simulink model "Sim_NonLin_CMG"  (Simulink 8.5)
settings: Solver=ode4  StartTime=0.0  StopTime=1800  FixedStep=Ts*1  RelTol=1e-3
InitFcn:
  | start
StopFcn:
  | Pl2
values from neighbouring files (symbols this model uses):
  Ave = [    [vehicle_flex34.m]    (also in vehicle_rigid.m)
  Bve = [    [vehicle_flex34.m]    (also in vehicle_rigid.m)
  CB2L = [cpsi, -cphi*spsi,  sphi*spsi;          0,    cphi,      -sphi;          0,    sphi*cpsi,  cphi*cpsi]/cpsi    [Rigbod_Dynam_LVLH.m]    (also in start.m = eye(3); start2.m = eye(3); start3.m = eye(3); start1.m = eye(3))
  com_dir = com_dir/sqrt(com_dir'*com_dir)    [start.m]    (also in start2.m; start3.m; start1.m)
  Cve = [    [vehicle_flex34.m]    (also in vehicle_rigid.m)
  d2r = pi/180    (= 0.0174532925199)    [start.m]    (also in start2.m; start3.m; Dead_Band_DF.m; start1.m)
  Dve = [    [vehicle_flex34.m]    (also in vehicle_rigid.m)
  ini = [wbo; atto; Hco]    [start.m]    (also in start2.m; start3.m; start1.m)
  J = [0.119416e9, -0.476e7,   -0.1216e7;     -0.476e7,     0.40408e8, -0.30121e6;     -0.1216e7,   -0.30121e6,  0.110166e9]    [start.m]    (also in start2.m; start3.m; start1.m)
  KshC = 2*Wdot_Lim_CMG/WlimC    [start.m]    (also in start2.m; start3.m; start1.m)
  nt = 12    [start.m]    (also in start2.m; start3.m; start1.m)
  omg = 20*wo    (= 0.022)    [start.m]    (also in start2.m; start3.m; start1.m)
  r2d = 180/pi    (= 57.2957795131)    [start.m]    (also in start2.m; start3.m; start1.m)
  thecmd = 20    [start.m]    (also in start2.m; start3.m; start1.m = 0.1)
  Wdot_Lim_CMG = 0.0001*d2r    (= 1.74532925199e-06)    [start.m]    (also in start2.m; start3.m; start1.m)
  Wlim_CMG = 0.01*d2r    (= 0.000174532925199)    [start.m]    (also in start2.m; start3.m; start1.m)
  wo = 0.0011    [start.m]    (also in start2.m; start3.m; start1.m)
  zeb = 0.95    [start.m]    (also in start2.m; start3.m; start1.m)
undefined symbols (not defined in the file or in its folder): Rigbod_Dynam_LVLH, Torq_Lim, Wlim

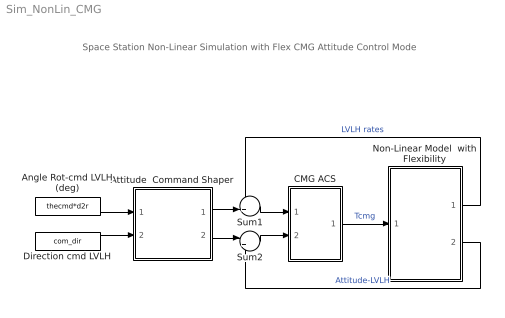
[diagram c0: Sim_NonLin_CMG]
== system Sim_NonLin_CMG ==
  note: Space Station Non-Linear Simulation with Flex CMG Attitude Control Mode
  Angle Rot-cmd LVLH (deg) : Constant  Value=thecmd*d2r
  Attitude  Command Shaper : Subsystem
  CMG ACS : Subsystem
  Direction cmd LVLH : Constant  Value=com_dir
  Non-Linear Model  with Flexibility : Subsystem
  Sum1 : Sum  Inputs=-+|
  Sum2 : Sum  Inputs=|+-
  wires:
  Non-Linear Model  with Flexibility/2(atti) -> Sum2/2  "Attitude-LVLH"
  Sum2/1 -> CMG ACS/2(ater)
  Non-Linear Model  with Flexibility/1(wlv) -> Sum1/1  "LVLH rates"
  Direction cmd LVLH/1 -> Attitude  Command Shaper/2(dir)
  Angle Rot-cmd LVLH (deg)/1 -> Attitude  Command Shaper/1(cmd)
  Sum1/1 -> CMG ACS/1(wl)
  CMG ACS/1(Tq) -> Non-Linear Model  with Flexibility/1(Tcmg)  "Tcmg"
  Attitude  Command Shaper/2(att-cmd) -> Sum2/1
  Attitude  Command Shaper/1(w-cmd) -> Sum1/2

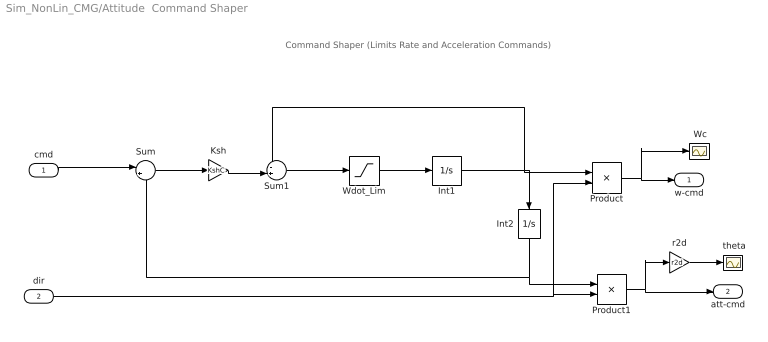
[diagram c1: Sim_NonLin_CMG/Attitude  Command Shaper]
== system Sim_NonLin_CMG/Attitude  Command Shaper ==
  note: Command Shaper (Limits Rate and Acceleration Commands)
  cmd : Inport  PortDimensions=1
  dir : Inport  Port=2  PortDimensions=3
  " Wc" : Scope
  " theta" : Scope
  Int1 : Integrator  LimitOutput=on  UpperSaturationLimit=Wlim_CMG  LowerSaturationLimit=-Wlim_CMG
  Int2 : Integrator  UpperSaturationLimit=Wlim  LowerSaturationLimit=-Wlim
  Ksh : Gain  Gain=KshC
  Product : Product
  Product1 : Product
  Sum : Sum  Inputs=|+-
  Sum1 : Sum  Inputs=-+|
  Wdot_Lim : Saturate  UpperLimit=Wdot_Lim_CMG  LowerLimit=-Wdot_Lim_CMG
  r2d : Gain  Gain=r2d
  w-cmd : Outport  PortDimensions=3
  att-cmd : Outport  Port=2  PortDimensions=3
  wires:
  Wdot_Lim/1 -> Int1/1
  Sum1/1 -> Wdot_Lim/1
  Int1/1 -> Product/1, Sum1/1, Int2/1
  Sum/1 -> Ksh/1
  Ksh/1 -> Sum1/2
  Int2/1 -> Sum/2, Product1/1
  cmd/1 -> Sum/1
  dir/1 -> Product/2, Product1/2
  r2d/1 -> " theta"/1
  Product/1 -> w-cmd/1, " Wc"/1
  Product1/1 -> att-cmd/1, r2d/1

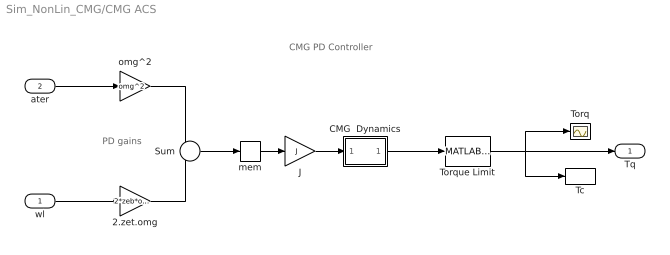
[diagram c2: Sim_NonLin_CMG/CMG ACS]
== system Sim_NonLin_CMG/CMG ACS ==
  note: CMG PD Controller
  note: PD gains
  wl : Inport
  ater : Inport  Port=2  PortDimensions=3
  2.zet.omg : Gain  Gain=2*zeb*omg
  CMG  Dynamics : Subsystem
  J : Gain  Gain=J  Multiplication=Matrix(K*u)
  Sum : Sum  Inputs=--
  Tc : ToWorkspace  VariableName=Tcmg  SampleTime=-1
  Torq : Scope
  Torque Limit : MATLABFcn  MATLABFcn=Torq_Lim( u(1:3) )  OutputDimensions=3
  mem : Memory
  omg^2 : Gain  Gain=omg^2
  Tq : Outport
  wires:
  wl/1 -> 2.zet.omg/1
  Sum/1 -> mem/1
  2.zet.omg/1 -> Sum/2
  ater/1 -> omg^2/1
  omg^2/1 -> Sum/1
  J/1 -> CMG  Dynamics/1(I)
  mem/1 -> J/1
  Torque Limit/1 -> Tq/1, Torq/1, Tc/1
  CMG  Dynamics/1(O) -> Torque Limit/1

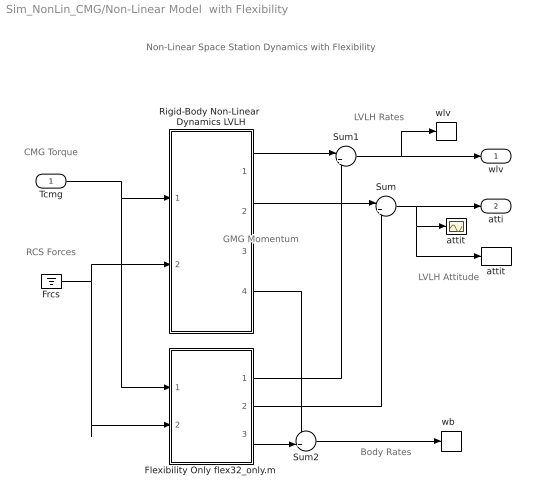
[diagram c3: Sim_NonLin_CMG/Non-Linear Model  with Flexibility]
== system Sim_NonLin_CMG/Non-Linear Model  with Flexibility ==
  note: Non-Linear Space Station Dynamics with Flexibility
  note: LVLH Attitude
  note: Body Rates
  note: RCS Forces
  note: CMG Torque
  note: LVLH Rates
  note: GMG Momentum
  Tcmg : Inport
  " attit " : Scope
  Flexibility Only flex32_only.m : Subsystem
  Frcs : Ground
  Rigid-Body Non-Linear  Dynamics LVLH : Subsystem
  Sum : Sum  Inputs=|++
  Sum1 : Sum  Inputs=|++
  Sum2 : Sum  Inputs=++|
  attit : ToWorkspace  VariableName=theta  SampleTime=-1
  "wb  " : ToWorkspace  VariableName=wb  SampleTime=-1
  "wlv  " : ToWorkspace  VariableName=wl  SampleTime=-1
  wlv : Outport
  atti : Outport  Port=2
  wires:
  Frcs/1 -> Rigid-Body Non-Linear  Dynamics LVLH/2(Frcs), Flexibility Only flex32_only.m/2(Frcs)
  Rigid-Body Non-Linear  Dynamics LVLH/2(atti-lv) -> Sum/1
  Flexibility Only flex32_only.m/2(att) -> Sum/2
  Sum/1 -> atti/1, " attit "/1, attit/1
  Sum1/1 -> wlv/1, "wlv  "/1
  Tcmg/1 -> Rigid-Body Non-Linear  Dynamics LVLH/1(Tcmg), Flexibility Only flex32_only.m/1(Tcmg)
  Rigid-Body Non-Linear  Dynamics LVLH/1(w-lv) -> Sum1/1
  Flexibility Only flex32_only.m/1(wbf) -> Sum1/2
  Flexibility Only flex32_only.m/3(wb) -> Sum2/2
  Rigid-Body Non-Linear  Dynamics LVLH/4(wb) -> Sum2/1
  Sum2/1 -> "wb  "/1

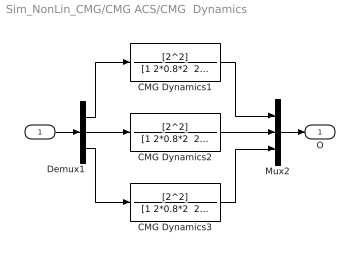
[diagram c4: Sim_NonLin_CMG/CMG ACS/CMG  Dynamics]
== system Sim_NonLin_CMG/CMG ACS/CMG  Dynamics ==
  I : Inport
  CMG Dynamics1 : TransferFcn  Numerator=[2^2]  Denominator="[1 2*0.8*2  2^2]"
  CMG Dynamics2 : TransferFcn  Numerator=[2^2]  Denominator="[1 2*0.8*2  2^2]"
  CMG Dynamics3 : TransferFcn  Numerator=[2^2]  Denominator="[1 2*0.8*2  2^2]"
  Demux1 : Demux  Outputs=3
  Mux2 : Mux  Inputs=3
  O : Outport
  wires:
  Mux2/1 -> O/1
  I/1 -> Demux1/1
  Demux1/3 -> CMG Dynamics3/1
  Demux1/1 -> CMG Dynamics1/1
  Demux1/2 -> CMG Dynamics2/1
  CMG Dynamics1/1 -> Mux2/1
  CMG Dynamics3/1 -> Mux2/3
  CMG Dynamics2/1 -> Mux2/2

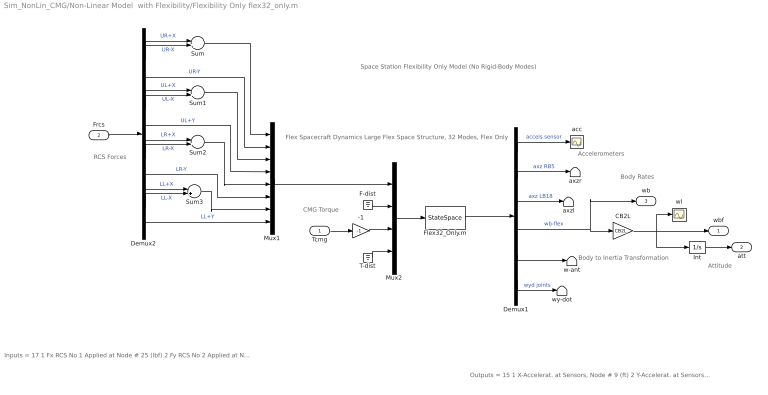
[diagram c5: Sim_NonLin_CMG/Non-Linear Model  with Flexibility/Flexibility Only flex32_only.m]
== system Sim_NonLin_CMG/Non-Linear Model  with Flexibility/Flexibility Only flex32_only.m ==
  note: Space Station Flexibility Only Model (No Rigid-Body Modes)
  note: Body to Inertia Transformation
  note: Attitude
  note: Body Rates
  note: Accelerometers
  note: Flex Spacecraft Dynamics Large Flex Space Structure, 32 Modes, Flex Only
  note: CMG Torque
  note: RCS Forces
  note: Inputs = 17 1 Fx RCS No 1 Applied at Node # 25 (lbf) 2 Fy RCS No 2 Applied at Node # 25 (lbf) 3 Fx RCS No 3 Applied at Node # 26 (lbf) 4 Fy RCS No 4 Applied at Node # 26 (lbf) 5 Fx RCS No 5 Applied at Node # 27 (lbf) 6 Fy RCS No 6 Applied at Node # 27 (lbf) 7 Fx RCS No 7 Applied at Node # 28 (lbf) 8 Fy RCS No 8 Applied at Node # 28 (lbf) 9 Fx Disturb. No 9 at Node # 21 (lbf) 10 Fy Disturb. No 10 at Node # 21 (lbf) 11 Fz Disturb. No 11 at Node # 21 (lbf) 12 Torq-x No 1 CMG Applied at Node # 10 (ft-lb) 13 Torq-y No 2 CMG Applied at Node # 10 (ft-lb) 14 Torq-z No 3 CMG Applied at Node # 10 (ft-lb) 15 Torq-x No 4 Gimbal Dist. at Node # 1 (ft-lb) 16 Torq-y No 5 Gimbal Dist. at Node # 1 (ft-lb) 17 Torq-z No 6 Gimbal Dist. at Node # 1 (ft-lb)
  note: Outputs = 15 1 X-Accelerat. at Sensors, Node # 9 (ft) 2 Y-Accelerat. at Sensors, Node # 9 (ft) 3 Z-Accelerat. at Sensors, Node # 9 (ft) 4 X-Accelerat. at Right Boom End, Node # 5 (ft) 5 Z-Accelerat. at Right Boom End, Node # 5 (ft) 6 X-Accelerat. at Left Boom End, Node # 18 (ft) 7 Z-Accelerat. at Left Boom End, Node # 18 (ft) 8 X-Rot. Rate at Sensors, Node # 9 (radian) 9 Y-Rot. Rate at Sensors, Node # 9 (radian) 10 Z-Rot. Rate at Sensors, Node # 9 (radian) 11 X-Rot. Rate at Antena Bot-Left, Node # 24 (radian) 12 Y-Rot. Rate at Antena Bot-Left, Node # 24 (radian) 13 Z-Rot. Rate at Antena Bot-Left, Node # 24 (radian) 14 Y-Rot.Accel. at Right Joint, Node # 7 (radian) 15 Y-Rot.Accel. at Left Joint, Node # 16 (radian)
  Tcmg : Inport
  Frcs : Inport  Port=2
  -1 : Gain  Gain=-1
  CB2L : Gain  Gain=CB2L  Multiplication=Matrix(K*u)
  Demux1 : Demux  Outputs=[3, 2, 2, 3, 3, 2]
  Demux2 : Demux  Outputs=12
  F-dist : Ground
  Flex32_Only.m : StateSpace  A=Ave  B=Bve  C=Cve  D=Dve  X0=0
  Int : Integrator
  Mux1 : Mux  Inputs=8
  Mux2 : Mux  Inputs=[8, 3, 3, 3]
  Sum{,1..3} (4 alike) : Sum  Inputs=|+-
  T-dist : Ground
  acc : Scope
  axzl : Terminator
  axzr : Terminator
  w-ant : Terminator
  wl : Scope
  wy-dot : Terminator
  wbf : Outport
  att : Outport  Port=2
  wb : Outport  Port=3
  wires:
  Demux1/6 -> wy-dot/1  "wyd joints"
  Demux1/5 -> w-ant/1
  T-dist/1 -> Mux2/4
  F-dist/1 -> Mux2/2
  Demux1/3 -> axzl/1  "axz LB18"
  Demux1/2 -> axzr/1  "axz RB5"
  Tcmg/1 -> -1/1
  Demux1/4 -> CB2L/1, wb/1  "wb-flex"
  Demux1/1 -> acc/1  "accels sensor"
  Flex32_Only.m/1 -> Demux1/1
  Mux2/1 -> Flex32_Only.m/1
  Mux1/1 -> Mux2/1
  Frcs/1 -> Demux2/1
  Demux2/6 -> Mux1/4  "UL+Y"
  Demux2/9 -> Mux1/6  "LR-Y"
  Demux2/12 -> Mux1/8  "LL+Y"
  Demux2/3 -> Mux1/2  "UR-Y"
  Demux2/1 -> Sum/1  "UR+X"
  Demux2/2 -> Sum/2  "UR-X"
  Sum/1 -> Mux1/1
  Demux2/4 -> Sum1/1  "UL+X"
  Demux2/5 -> Sum1/2  "UL-X"
  Sum1/1 -> Mux1/3
  Demux2/7 -> Sum2/1  "LR+X"
  Demux2/8 -> Sum2/2  "LR-X"
  Demux2/10 -> Sum3/1  "LL+X"
  Demux2/11 -> Sum3/2  "LL-X"
  Sum3/1 -> Mux1/7
  Sum2/1 -> Mux1/5
  Int/1 -> att/1
  -1/1 -> Mux2/3
  CB2L/1 -> wl/1, wbf/1, Int/1

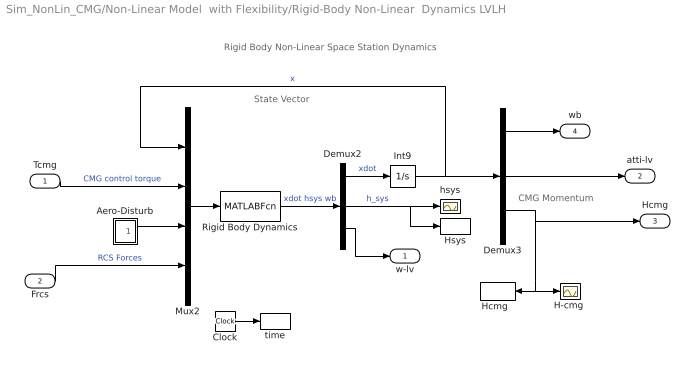
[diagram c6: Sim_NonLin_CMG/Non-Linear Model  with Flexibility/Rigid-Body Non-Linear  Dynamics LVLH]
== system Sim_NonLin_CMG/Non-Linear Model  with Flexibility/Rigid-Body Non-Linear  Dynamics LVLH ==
  note: CMG Momentum
  note: State Vector
  note: Rigid Body Non-Linear Space Station Dynamics
  Tcmg : Inport  PortDimensions=3
  Frcs : Inport  Port=2  PortDimensions=nt
  Aero-Disturb : Subsystem
  Clock : Clock
  Demux2 : Demux  Outputs=[9,3,3]
  Demux3 : Demux  Outputs=[3,3,3]
  "H-cmg " : Scope
  "Hcmg  " : ToWorkspace  VariableName=Hcmg  SampleTime=-1
  Hsys : ToWorkspace  VariableName=Hsys  SampleTime=-1
  Int9 : Integrator  InitialCondition=ini
  Mux2 : Mux  Inputs=[9, 3, 3, nt]
  Rigid Body Dynamics : MATLABFcn  MATLABFcn=Rigbod_Dynam_LVLH( u(1:9), u(10:12), u(13:15), u(16:15+nt) )  OutputDimensions=15
  hsys : Scope
  time : ToWorkspace  VariableName=time  SampleTime=-1
  w-lv : Outport
  atti-lv : Outport  Port=2
  Hcmg : Outport  Port=3
  wb : Outport  Port=4
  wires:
  Mux2/1 -> Rigid Body Dynamics/1
  Clock/1 -> time/1
  Frcs/1 -> Mux2/4  "RCS Forces"
  Demux3/3 -> Hcmg/1, "H-cmg "/1, "Hcmg  "/1
  Demux3/2 -> atti-lv/1
  Demux2/2 -> Hsys/1, hsys/1  "h_sys"
  Demux2/3 -> w-lv/1
  Tcmg/1 -> Mux2/2  "CMG control torque"
  Int9/1 -> Mux2/1, Demux3/1  "x"
  Demux2/1 -> Int9/1  "xdot"
  Rigid Body Dynamics/1 -> Demux2/1  "xdot hsys wb"
  Aero-Disturb/1(Td) -> Mux2/3
  Demux3/1 -> wb/1

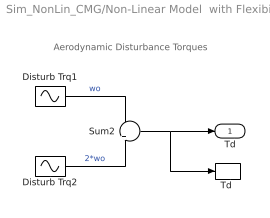
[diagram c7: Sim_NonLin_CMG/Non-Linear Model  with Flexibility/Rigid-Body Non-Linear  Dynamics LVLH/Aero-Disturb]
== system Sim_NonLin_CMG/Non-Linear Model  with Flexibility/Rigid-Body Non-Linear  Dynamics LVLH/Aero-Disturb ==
  note: Aerodynamic Disturbance Torques
  Disturb Trq1 : Sin  Amplitude=[1, 3, 1]  Bias="[1  8  1]"  Frequency=[wo, wo, wo]  SampleTime=0
  Disturb Trq2 : Sin  Amplitude=[1, 1, 1]*0.5  Frequency=[wo, wo, wo]*2  SampleTime=0
  Sum2 : Sum  Inputs=+|+
  "Td " : ToWorkspace  VariableName=Td  SampleTime=-1
  Td : Outport
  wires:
  Disturb Trq2/1 -> Sum2/2  "2*wo"
  Sum2/1 -> "Td "/1, Td/1
  Disturb Trq1/1 -> Sum2/1  "wo"
